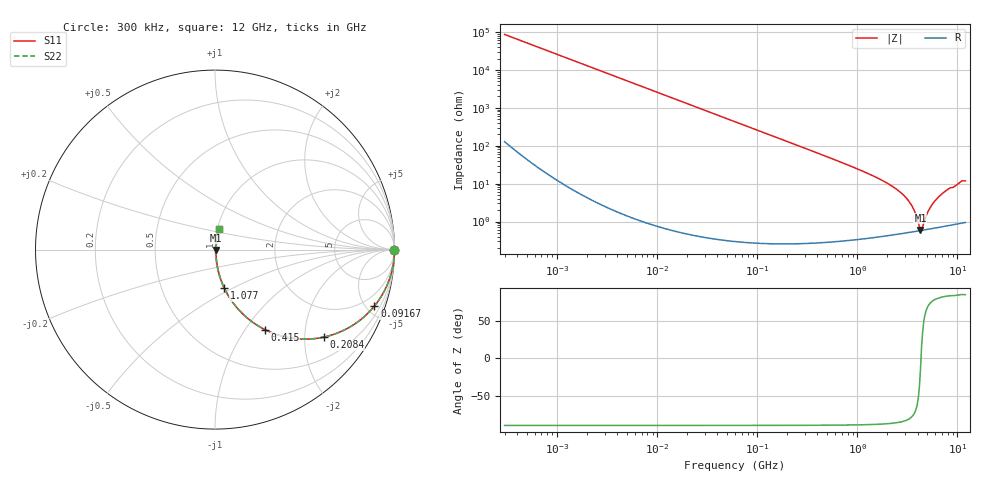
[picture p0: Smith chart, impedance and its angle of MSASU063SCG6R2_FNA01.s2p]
! MSASU063SCG6R2_FNA01  S-PARAMETER MODEL  ( Standard Model )
! Model Generated by TAIYO YUDEN Corporation (http://www.ty-top.com)
! Version 1.0
! TAIYO YUDEN Control No. 240819
! Copyright(c) 2024 TAIYO YUDEN CO.,LTD. All Rights Reserved.
! Product Description (link to TY-COMPAS)
! https://ds.yuden.co.jp/TYCOMPAS/or/detail?pn=MSASU063SCG6R2DFNA01&u=M
! Products Name : Multilayer Ceramic Capacitors
! Characteristics :
!  Capacitance : 6.2 [pF] , Rated Voltage : 50 [V] , TCC : CG / C0G
!  Case Size : 0.6 x 0.3 / 0.024 x 0.012 [mm/inch] , Thickness : 0.3 / 0.012 [mm/inch]
!  (Conditions: Temperature = 25 [degC] , DC Bias Voltage = 0 [V])
! External Node Assignments :
!  1  o---| |---o  2
! GND o---------o GND
! Frequency Range : 0.3MHz  -  12000MHz  [ 401 STEP ]
# MHZ S RI R 50
! Freq[MHz].  S11 Real  S11 Imag  S21 Real  S21 Imag  S12 Real  S12 Imag  S22 Real  S22 Imag
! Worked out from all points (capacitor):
!   401 points, 300 kHz to 12 GHz, reference 50 ohm
!   read as one part in series: C = 6.15 pF near 316.3 kHz
!   lowest |Z| = 597 mohm at 4.271 GHz (marker M1)
!   series resonance near 4.324 GHz, so ESL is about 220 pH
!   S11 on the Smith chart (normalised r, x): 300 kHz: open; 91.67 MHz: 1.01, -5.64; 208.4 MHz: 1.01, -2.48; 415 MHz: 1.01, -1.24; 1.077 GHz: 1.01, -0.45; 12 GHz: 1.02, +0.24
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0.3  1 -0.00116  3.06e-06 0.00116  3.06e-06 0.00116  1 -0.00116
1.769972  1 -0.00684  4.92e-05 0.00684  4.92e-05 0.00684  1 -0.00684
10.44266  0.9984 -0.0403  0.00164 0.0403  0.00164 0.0403  0.9984 -0.0403
27.82928  0.9885 -0.1063  0.0115 0.1063  0.0115 0.1063  0.9885 -0.1063
60  0.9488 -0.2201  0.0512 0.2201  0.0512 0.2201  0.9488 -0.2201
91.67136  0.8881 -0.3148  0.1119 0.3148  0.1119 0.3148  0.8881 -0.3148
208.3979  0.6051 -0.4878  0.3949 0.4878  0.3949 0.4878  0.6051 -0.4878
353.9943  0.3456 -0.4737  0.6544 0.4737  0.6544 0.4737  0.3456 -0.4737
414.98  0.277 -0.4453  0.723 0.4453  0.723 0.4453  0.277 -0.4453
651.0506  0.133 -0.3357  0.867 0.3357  0.867 0.3357  0.133 -0.3357
1076.992  0.0512 -0.2131  0.9488 0.2131  0.9488 0.2131  0.0512 -0.2131
2088.533  0.0131 -0.0934  0.9869 0.0934  0.9869 0.0934  0.0131 -0.0934
2722.03  0.00798 -0.0567  0.992 0.0567  0.992 0.0567  0.00798 -0.0567
3276.641  0.00623 -0.0333  0.9938 0.0333  0.9938 0.0333  0.00623 -0.0333
3642.919  0.00577 -0.0205  0.9942 0.0205  0.9942 0.0205  0.00577 -0.0205
4270.516  0.00573 -0.00153  0.9943 0.00153  0.9943 0.00153  0.00573 -0.00153
4502.883  0.00589 0.0044  0.9941 -0.0044  0.9941 -0.0044  0.00589 0.0044
5006.236  0.0064 0.0154  0.9936 -0.0154  0.9936 -0.0154  0.0064 0.0154
5420.343  0.00696 0.0239  0.993 -0.0239  0.993 -0.0239  0.00696 0.0239
6354.153  0.00857 0.041  0.9914 -0.041  0.9914 -0.041  0.00857 0.041
8064.993  0.0126 0.0695  0.9874 -0.0695  0.9874 -0.0695  0.0126 0.0695
12000  0.0227 0.114  0.9773 -0.114  0.9773 -0.114  0.0227 0.114
